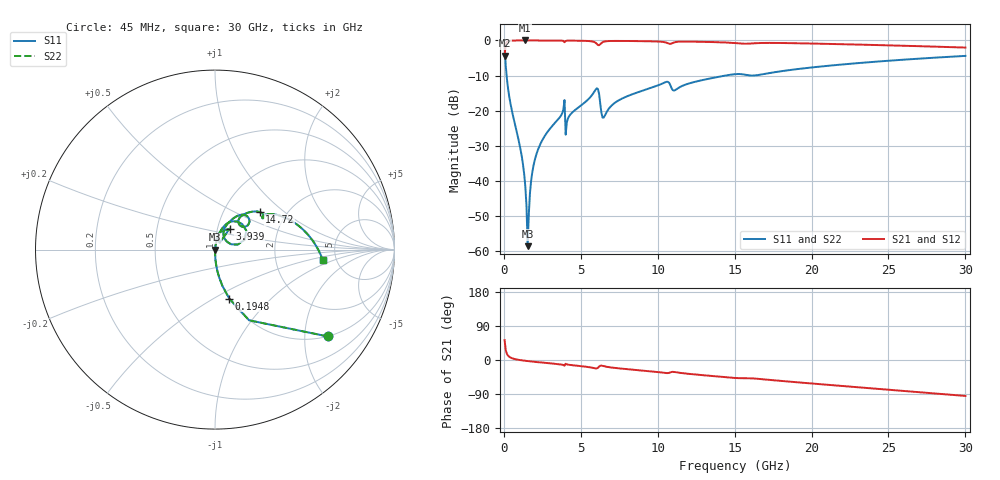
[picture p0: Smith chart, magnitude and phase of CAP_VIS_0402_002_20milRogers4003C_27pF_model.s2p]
! S-parameter model data by Modelithics Inc.  support@modelithics.com  813-866-6335  Tampa FL USA
! S-Parameter data specifications:
! Substrate: 20-mil Rogers 4003C, substrate thickness, H=0.508mm, Dielectric constant, Er=3.75
! PCB Mounting Pad Footprint: Pad width, PadW=0.50mm , Pad length, PadL=0.50mm , Pad gap, PadG (edge-to-edge)=0.40mm , Reference planes=1.4mm apart
! Created Wed Nov 18 12:53:26 2015
# hz S ma R 50
! 2 Port Network Data from SP1.SP block
! freq  magS11  angS11  magS21  angS21  magS12  angS12  magS22  angS22
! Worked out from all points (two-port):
!   401 points, 45 MHz to 30 GHz, reference 50 ohm
!   highest |S21| = -0.01 dB at 1.393 GHz (marker M1); lowest = -4.3 dB at 45 MHz (marker M2)
!   |S21| within 3 dB of the highest: 73.76 MHz to end of sweep
!   lowest |S11| = -58.5 dB at 1.543 GHz (marker M3), VSWR 1.00, Z = 50.1 - j0.0522 ohm
!   |S11| at or under -10 dB: 176.2 MHz to 14.4 GHz (14.22 GHz wide, 195 % of centre)
!   |S22| runs from -58.5 to -2.0 dB; largest |S21 - S12| = 0
!   S11 on the Smith chart (normalised r, x): 45 MHz: 1.00, -2.60; 194.8 MHz: 1.00, -0.59; 3.939 GHz: 1.14, +0.27; 14.72 GHz: 1.47, +0.69; 30 GHz: 3.90, -0.69
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4.5e7  0.7931 -37.6  0.6089 52.4  0.6089 52.4  0.7931 -37.6
1.94775e8  0.2842 -73.8  0.9584 16.1  0.9584 16.1  0.2842 -73.8
3.4455e8  0.1598 -81.3  0.9866 8.5  0.9866 8.5  0.1598 -81.3
1.168312e9  0.02186 -88.4  0.9988 -0.9  0.9988 -0.9  0.02186 -88.4
1.392975e9  0.00831 -85.0  0.9989 -2.1  0.9989 -2.1  0.00831 -85.0
1.54275e9  0.001184 -26.1  0.9989 -2.9  0.9989 -2.9  0.001184 -26.1
1.692525e9  0.006704 76.7  0.9988 -3.5  0.9988 -3.5  0.006704 76.7
1.917188e9  0.01632 81.2  0.9986 -4.5  0.9986 -4.5  0.01632 81.2
2.291625e9  0.03079 81.5  0.9981 -6.1  0.9981 -6.1  0.03079 81.5
3.789375e9  0.09189 75.3  0.9919 -12.4  0.9919 -12.4  0.09189 75.3
3.93915e9  0.1418 55.1  0.9427 -15.0  0.9427 -15.0  0.1418 55.1
4.163812e9  0.07779 75.4  0.9937 -12.2  0.9937 -12.2  0.07779 75.4
5.062462e9  0.1213 71.7  0.9885 -16.4  0.9885 -16.4  0.1213 71.7
6.036e9  0.2082 43.1  0.8949 -22.2  0.8949 -22.2  0.2082 43.1
6.560212e9  0.08516 53.5  0.9679 -16.9  0.9679 -16.9  0.08516 53.5
1.007992e10  0.2321 55.3  0.9626 -32.2  0.9626 -32.2  0.2321 55.3
1.112835e10  0.1962 47.7  0.9456 -31.9  0.9456 -31.9  0.1962 47.7
1.472295e10  0.3249 40.1  0.9262 -46.5  0.9262 -46.5  0.3249 40.1
1.50225e10  0.3309 37.9  0.9164 -47.4  0.9164 -47.4  0.3309 37.9
2.003996e10  0.4132 26.9  0.9028 -62.1  0.9028 -62.1  0.4132 26.9
2.505742e10  0.5152 10.8  0.8506 -78.6  0.8506 -78.6  0.5152 10.8
3e10  0.6024 -5.3  0.7914 -94.8  0.7914 -94.8  0.6024 -5.3
